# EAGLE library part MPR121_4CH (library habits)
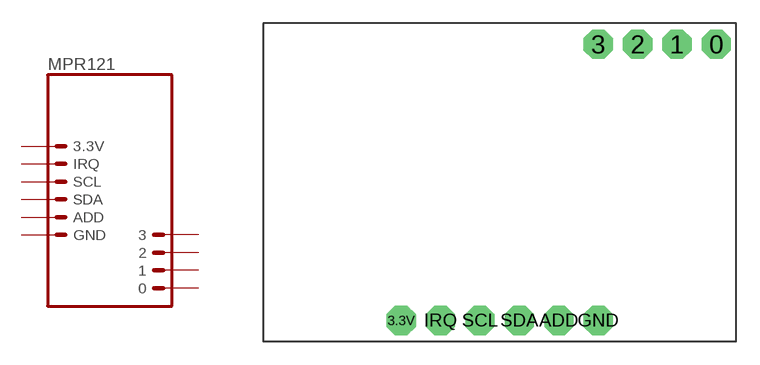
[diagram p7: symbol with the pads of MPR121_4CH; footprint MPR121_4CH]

Designator prefix U

## MPR121_4CH  [MPR121_4CH]
0  0  pas
1  1  pas
2  2  pas
3  3  pas
3.3V  3.3V  pas
ADD  ADD  pas
GND  GND  pas
IRQ  IRQ  pas
SCL  SCL  pas
SDA  SDA  pas

## Footprint MPR121_4CH (pad centres in mm)
Plated Through Hole - 2x12 Specifications: Pin count:24 Pin pitch:0.1" Example device(s): CONN_12x2
drill 1.016 pad 1.88 octagon: 0 13.97,8.9; 1 11.43,8.9; 2 8.89,8.9; 3 6.35,8.9; 3.3V -6.35,-8.9; ADD 3.81,-8.9; GND 6.35,-8.9; IRQ -3.81,-8.9; SCL -1.27,-8.9; SDA 1.27,-8.9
